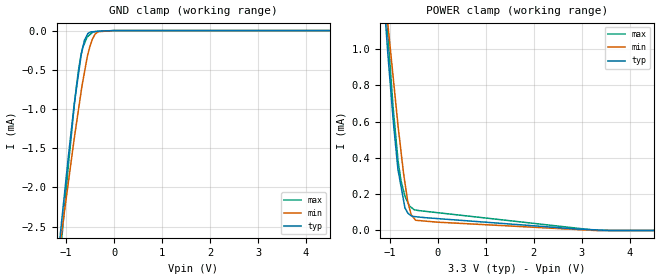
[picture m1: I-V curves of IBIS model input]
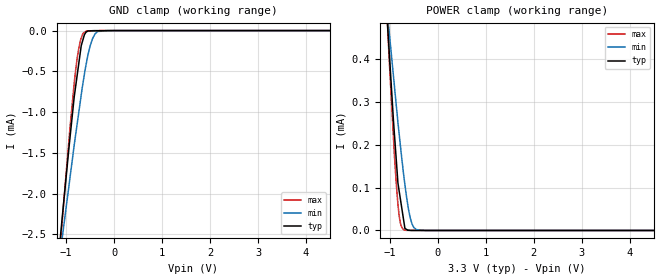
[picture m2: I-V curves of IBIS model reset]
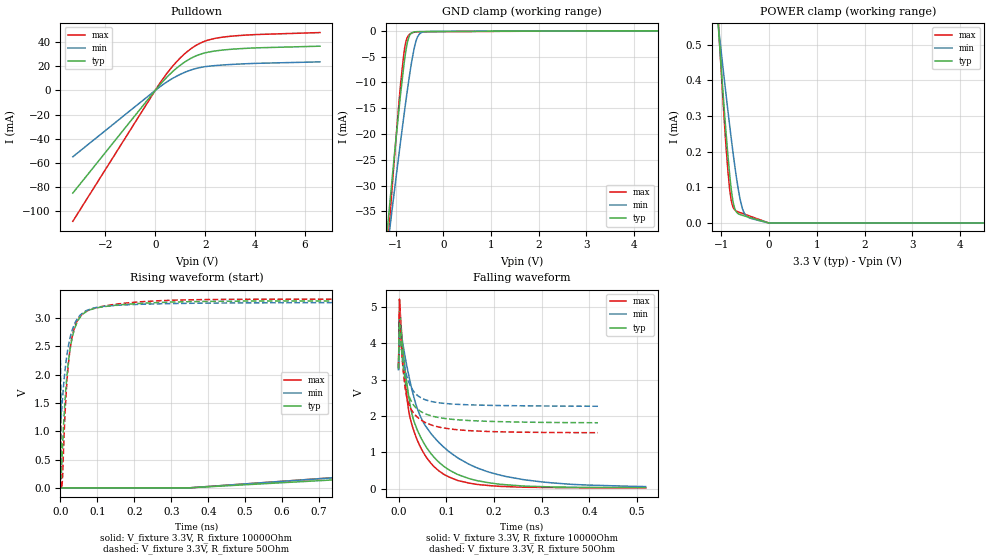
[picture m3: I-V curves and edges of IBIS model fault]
|Texas Instruments Incorporated
| 125W PurePath Digital-Input Class-D Power Stage
| Marketing part#   Digital Voltage Range   Package-type   #pins
| TAS5612LADDV   3.27V - 3.33V   DDV   44
[IBIS Ver]   3.2
[File name]   tas5612la.ibs
|SIMDE Ver   V3.0 - 201101 - Build 457
[File Rev]   1.0
[Date]   5/24/2012
[Source]
| Texas Instruments Incorporated.
| Analog-eLab Design Center, HPA
| 12500 TI Blvd
| Dallas, TX -75243
| e-mail: elab_scm_ibis@list.ti.com
[Notes]   Revision History:
| Rev 1.0: 5/24/2012
| - Initial version of the model
| - Model generated from simulations in TISPICE
| - Model matched to SPICE simulation
| - C_comp although listed in numerical order of value are
|   obtained from varying PVT conditions. For PVT conditions for
|   each specific value refer the buffer description under
|   respective [Model]. IBIS model user is responsible for using
|   appropriate C_comp to simulate for Signal Integrity.
| - Model names with a trailing _3p3 contains the model for
|   3.3V [3.27V and 3.33V].
|*  EXCEPTION:   *
|*  - For model fault, there will be a leakage current in the ground clamp  *
|*   I-V Table because of the pull-down transistor connected to pad.   *
|*  - For model clip_otw, there will be a leakage current in the ground   *
|*   clamp I-V Table because of the pull-down transistor connected to pad. *
|*  - For model input, there will be a leakage current in the power clamp   *
|*   I-V Table because of the series resistor connected to pad.   *
[Disclaimer]
| This model is designed as an aid for customers of Texas Instruments.
| TI and its licensors and suppliers make no warranties, either expressed
| or implied, with respect to this  model, including the warranties of
| merchantability or fitness for a particular purpose. The model is
| provided solely on an "as is" basis. The entire risk as to its quality
| and performance is with the customer.
[Copyright]
 (C) Copyright 2012 Texas Instruments Incorporated.All rights reserved.
|   TAS5612LA
[Component]   TAS5612LA
[Manufacturer]   TI
[Package]   |44 HTSSOP   -  DDV package
|   typ   min   max
R_pkg   0.01988   0.00761   0.02820
L_pkg   2.83543nH   1.88996nH   4.38501nH
C_pkg   0.51432pF   0.36166pF   0.71632pF
[Pin]  signal_name   model_name   R_pin   L_pin   C_pin
1   GVDD_AB   power   0.02936   5.14716nH  0.69484pF
2   VDD   power   0.02818   4.35374nH  0.68163pF
3   OC_ADJ   term   0.02761   3.69494nH  0.59541pF
4   _RESET   reset   0.02780   2.93180nH  0.42730pF
5   INPUT_A   term   0.02705   2.67858nH  0.37968pF
6   INPUT_B   term   0.02543   2.55669nH  0.37641pF
7   C_START   term   0.02324   2.39533nH  0.36233pF
8   DVDD   power   0.02065   2.21891nH  0.35477pF
9   GND   gnd   0.01893   2.09064nH  0.33358pF
10   GND   gnd   0.00713   1.79670nH  0.39618pF
11   GND   gnd   0.01384   2.26449nH  0.48602pF
12   GND   gnd   0.01381   2.27641nH  0.50323pF
13   AVDD   power   0.01424   2.33727nH  0.49485pF
14   INPUT_C   term   0.01450   2.38491nH  0.47685pF
15   INPUT_D   term   0.00761   1.88996nH  0.42531pF
16   _FAULT   fault   0.02194   2.31148nH  0.36166pF
17   _OTW   clip_otw   0.02528   2.56022nH  0.38380pF
18   _CLIP   clip_otw   0.02759   2.73531nH  0.38538pF
19   M1   input   0.02784   2.95107nH  0.42848pF
20   M2   input   0.02765   3.72216nH  0.59629pF
21   M3   input   0.02820   4.38501nH  0.67248pF
22   GVDD_CD   power   0.02952   5.32362nH  0.69982pF
23   BST_D   power   0.03232   5.58639nH  0.73537pF
24   BST_C   power   0.03291   4.81347nH  0.71048pF
25   GND   gnd   0.01175   2.94907nH  0.69322pF
26   GND   gnd   0.01186   3.22097nH  0.72361pF
27   OUT_D   term   0.01242   3.06871nH  0.71632pF
28   OUT_D   term   0.01136   2.96126nH  0.69613pF
29   PVDD_CD   power   0.01095   2.67072nH  0.66354pF
30   PVDD_CD   power   0.00938   2.40709nH  0.64271pF
31   PVDD_CD   power   0.00877   2.29583nH  0.58088pF
32   OUT_C   term   0.00921   2.31587nH  0.54265pF
33   GND   gnd   0.00969   2.46906nH  0.57388pF
34   GND   gnd   0.00969   2.46836nH  0.57309pF
35   OUT_B   term   0.00921   2.31539nH  0.54237pF
36   PVDD_AB   power   0.00878   2.29480nH  0.58034pF
37   PVDD_AB   power   0.00938   2.40544nH  0.64104pF
38   PVDD_AB   power   0.01095   2.66739nH  0.66097pF
39   OUT_A   term   0.01135   2.95115nH  0.68999pF
40   OUT_A   term   0.01242   3.06329nH  0.71322pF
41   GND   gnd   0.01186   3.16015nH  0.72229pF
42   GND   gnd   0.01174   2.94100nH  0.69314pF
43   BST_B   power   0.03289   4.77644nH  0.71393pF
44   BST_A   power   0.03229   5.53352nH  0.73759pF
[Model] term
Model_type Terminator
C_comp   1.0e-20F  1.0e-20F  1.0e-20F
|   typ   min   max
[Voltage Range]   3.3V   3.27V   3.33V
[POWER Clamp Reference]   3.3V   3.27V   3.33V
[GND Clamp Reference]   0V   0V   0V
|Ambient Temperature   25   70   0
|Junction Temperature
[Temperature Range]   27   125   0
| Models and submodels in the file (5): input (Input), reset (Input), fault (I/O_open_drain), clip_otw (Open_drain), term (Terminator)
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|   input Model
[Model]   input
Model_type   Input
Vinl = 0.8
Vinh = 1.9
|   typ   min   max
|   (nom PVT)   (fast PVT)   (slow PVT)
C_comp   2.383e-14   3.303e-15   3.538e-14
| Where nom  PVT is Nominal Process, 3.3V, 27C
|   Fast PVT is Strong Process,  3.33V, 0C
|   Slow PVT is Weak Process,   3.27V, 125C
[Voltage Range]   3.3   3.27   3.33
|Ambient Temperature   25   70   0
|Junction Temperature
[Temperature Range]   27   125   0
[Power Clamp Reference]   3.3   3.27   3.33
[GND Clamp Reference]   0   0   0
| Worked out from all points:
|   GND clamp passes 1 mA (typ) near -0.84 V on its own axis
|   POWER clamp passes 1 mA (typ) near -1.05 V on its own axis
[GND Clamp]
|   Voltage   I(typ)   I(min)   I(max)
-3.3V     -16.78mA   -13.25mA   -19.44mA
-1.112V   -2.542mA   -2.658mA   -2.794mA
-959mV    -1.641mA   -1.96mA    -1.755mA
-831.6mV  -942.3uA   -1.379mA   -961.1uA
-735.9mV  -525.1uA   -980.9uA   -482.8uA
-659.3mV  -234.9uA   -671.4uA   -227.1uA
-617.1mV  -122.2uA   -529.1uA   -162.5uA
-559.2mV  -52.14uA   -334uA     -81.21uA
-488.4mV  -16.8uA    -173.3uA   -43.59uA
-336.8mV  -9.061uA   -14.35uA   -11.13uA
-3.27mV   -64.82nA   -45.83nA   -96.5nA
6.6V      0A         0A         0A
[POWER Clamp]
|   Voltage   I(typ)   I(min)   I(max)
-3.3V     10.02mA    7.662mA    12.33mA
-1.125V   1.279mA    1.356mA    1.43mA
-1.056V   1.024mA    1.173mA    1.13mA
-1.04V    965.9uA    1.131mA    1.07mA
-932.4mV  612.3uA    848.3uA    677.8uA
-831.6mV  337.2uA    582.3uA    390.7uA
-769.2mV  246uA      439.1uA    275.6uA
-686.4mV  125uA      264.2uA    190.5uA
-627.8mV  96.81uA    160.6uA    155.5uA
-461.1mV  75.94uA    56.22uA    112.7uA
3.327V    2.999uA    0A         98nA
6.6V      0A         0A         0A
|   reset Model
[Model]   reset
Model_type   Input
Vinl = 0.8
Vinh = 1.9
|   typ   min   max
|   (nom PVT)   (fast PVT)   (slow PVT)
C_comp   2.377e-14   3.303e-15   3.567e-14
| Where nom  PVT is Nominal Process, 3.3V, 27C
|   Fast PVT is Strong Process,  3.33V, 0C
|   Slow PVT is Weak Process,   3.27V, 125C
[Voltage Range]   3.3   3.27   3.33
|Ambient Temperature   25   70   0
|Junction Temperature
[Temperature Range]   27   125   0
[Power Clamp Reference]   3.3   3.27   3.33
[GND Clamp Reference]   0   0   0
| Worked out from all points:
|   GND clamp passes 1 mA (typ) near -0.86 V on its own axis
|   POWER clamp passes 1 mA (typ) near -1.31 V on its own axis
[GND Clamp]
|   Voltage   I(typ)   I(min)   I(max)
-3.3V     -16.81mA   -13.3mA    -19.47mA
-1.154V   -2.754mA   -2.885mA   -2.878mA
-1.082V   -2.301mA   -2.549mA   -2.348mA
-1.042V   -2.056mA   -2.365mA   -2.053mA
-915.7mV  -1.294mA   -1.789mA   -1.17mA
-831.6mV  -814.3uA   -1.405mA   -645.7uA
-769.2mV  -546.4uA   -1.143mA   -338.1uA
-683.1mV  -181.5uA   -780.5uA   -86.66uA
-576.1mV  -16.4uA    -393.2uA   -4.834uA
-451.3mV  -3.585uA   -102.3uA   -1.308uA
-340.1mV  -2.374uA   -10.37uA   -20.25nA
6.6V      0A         0A         0A
[POWER Clamp]
|   Voltage   I(typ)   I(min)   I(max)
-3.3V     5.16mA     3.356mA    6.154mA
-1.049V   481.6uA    504.3uA    480.7uA
-1.016V   420.4uA    465.2uA    402.8uA
-905.8mV  225.7uA    337.7uA    176.3uA
-865.8mV  163.5uA    291.4uA    107.8uA
-829.2mV  108.5uA    249uA      57.64uA
-765.9mV  62.5uA     182.4uA    11.19uA
-689.3mV  6.826uA    109.7uA    815.9nA
-575.5mV  284.2nA    29.36uA    207.5nA
-500.3mV  47.55nA    6.964uA    115.3nA
-444.7mV  40.57nA    1.935uA    47.19nA
6.6V      0A         0A         0A
|   fault Model
[Model]   fault
Model_type   I/O_open_drain
Polarity   Inverting
Vinl = 0.8
Vinh = 1.9
Vmeas = 1.65
Vref = 3.3
Cref = 2pF
Rref = 10000
|   typ   min   max
|   (nom PVT)   (fast PVT)   (slow PVT)
C_comp   8.474e-13   8.413e-13   8.728e-13
|ON state : BUFFER OUTPUT TURNED LOW
|C_comp   8.474e-13   8.413e-13   8.728e-13
|OFF state: BUFFER IN HIGH IMPEDANCE
|C_comp   3.420e-13   2.951e-13   3.808e-13
| Where nom  PVT is Nominal Process, 3.3V, 27C
|   Fast PVT is Strong Process,  3.33V, 0C
|   Slow PVT is Weak Process,   3.27V, 125C
[Voltage Range]   3.3   3.27   3.33
|Ambient Temperature   25   70   0
|Junction Temperature
[Temperature Range]   27   125   0
[Pullup Reference]   3.3   3.27   3.33
[Pulldown Reference]   0   0   0
[Power Clamp Reference]   3.3   3.27   3.33
[GND Clamp Reference]   0   0   0
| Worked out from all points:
|   slope of the pulldown table from 0 to 0.495 V, typ, clamps not added: 42.9 ohm
|   GND clamp passes 1 mA (typ) near -0.71 V on its own axis
|   POWER clamp passes 1 mA (typ) near -1.29 V on its own axis
|   falling waveform, V_fixture 3.3V, R_fixture 10000Ohm: 20-80 % time 68.6ps typ, 114ps min, 52.7ps max; typ from 3.3 V to 0.024 V
|   rising waveform, V_fixture 3.3V, R_fixture 10000Ohm: 20-80 % time 6.39ns typ, 7.34ns min, 5.5ns max; typ from 0.018 V to 3.3 V
|   falling waveform, V_fixture 3.3V, R_fixture 50Ohm: 20-80 % time 34.3ps typ, 34.1ps min, 34.2ps max; typ from 3.3 V to 1.81 V
|   rising waveform, V_fixture 3.3V, R_fixture 50Ohm: 20-80 % time 32.9ps typ, 36.3ps min, 29.8ps max; typ from 1.8 V to 3.3 V
[Pulldown]
|   Voltage   I(typ)   I(min)   I(max)
-3.3V     -85.03mA   -54.97mA   -108.4mA
202.2mV   5.008mA    3.215mA    6.411mA
584.8mV   13.4mA     8.582mA    17.2mA
867.9mV   18.66mA    11.93mA    24.02mA
1.15V     23.07mA    14.72mA    29.81mA
1.432V    26.62mA    16.95mA    34.54mA
1.713V    29.29mA    18.6mA     38.22mA
1.995V    31.12mA    19.69mA    40.86mA
2.7V      33.45mA    21.07mA    44.13mA
3.969V    35.2mA     22.38mA    46.22mA
6.6V      36.67mA    23.68mA    47.95mA
[GND Clamp]
|   Voltage   I(typ)   I(min)   I(max)
-3.3V     -221mA     -192.5mA   -255.7mA
-1.802V   -99.82mA   -89.99mA   -119.1mA
-1.046V   -25.87mA   -32.43mA   -26.92mA
-914.1mV  -13.67mA   -22.63mA   -12.02mA
-825mV    -6.409mA   -16.25mA   -4.129mA
-785.9mV  -3.828mA   -13.55mA   -2.094mA
-742.9mV  -1.798mA   -10.69mA   -1.04mA
-654.6mV  -359.9uA   -5.418mA   -382.3uA
-594mV    -191.5uA   -2.644mA   -247.2uA
-542.8mV  -155.9uA   -1.179mA   -204.5uA
-402.6mV  -142.5uA   -182uA     -180uA
6.6V      0A         0A         0A
[POWER Clamp]
|   Voltage   I(typ)   I(min)   I(max)
-3.3V     5.287mA    3.463mA    6.313mA
-1.129V   677.4uA    632.8uA    715.7uA
-1.043V   509.2uA    527.2uA    513.6uA
-917.4mV  278.2uA    377.1uA    242.4uA
-825mV    133.2uA    271.4uA    92.66uA
-749.2mV  55.36uA    190.1uA    42.61uA
-697.1mV  33.33uA    138.8uA    34.64uA
-619.3mV  24.38uA    74.48uA    29.88uA
-542.8mV  20.92uA    34.29uA    26.13uA
-474.7mV  18.27uA    19.38uA    22.85uA
-570uV    21.98nA    19.17nA    93.78nA
6.6V      0A         0A         0A
[Ramp]
R_load = 10000
|   typ   min   max
dV/dt_r   1.96937/6.39593e-09   1.94632/7.34644e-09   1.98902/5.50141e-09
dV/dt_f   1.96937/6.89404e-11   1.94632/1.1684e-10   1.98902/5.28355e-11
[Falling Waveform]
V_fixture = 3.3V
V_fixture_min = 3.27V
V_fixture_max = 3.33V
R_fixture = 10000Ohm
|   Time   V(typ)   V(min)   V(max)
0s        3.3V       3.27V      3.33V
2ps       4.872V     4.615V     5.213V
8ps       3.997V     4.077V     3.995V
16ps      3.054V     3.472V     2.7V
26ps      2.185V     2.844V     1.86V
52ps      1.276V     1.822V     993.4mV
100ps     563.6mV    1.08V      355.2mV
152ps     258.2mV    642.1mV    139.7mV
226ps     103.4mV    329mV      52.78mV
518ps     23.99mV    53.6mV     18.42mV
[Rising Waveform]
V_fixture = 3.3V
V_fixture_min = 3.27V
V_fixture_max = 3.33V
R_fixture = 10000Ohm
|   Time   V(typ)   V(min)   V(max)
0s        17.72mV    26.13mV    14.97mV
348ps     0V         0V         0V
980ps     227.3mV    288.6mV    291.2mV
2.058ns   922.7mV    860.1mV    1.071V
4.398ns   1.828V     1.69V      2.048V
6.466ns   2.369V     2.201V     2.579V
9.208ns   2.797V     2.644V     2.961V
13.18ns   3.094V     2.983V     3.197V
16.9ns    3.208V     3.133V     3.282V
35ns      3.3V       3.27V      3.33V
[Falling Waveform]
V_fixture = 3.3V
V_fixture_min = 3.27V
V_fixture_max = 3.33V
R_fixture = 50Ohm
|   Time   V(typ)   V(min)   V(max)
0s        3.3V       3.27V      3.33V
2ps       4.574V     4.335V     4.875V
4ps       4.18V      4.08V      4.328V
8ps       3.585V     3.68V      3.513V
12ps      3.161V     3.381V     2.957V
16ps      2.854V     3.155V     2.594V
28ps      2.368V     2.749V     2.144V
50ps      2.096V     2.478V     1.862V
146ps     1.873V     2.305V     1.595V
418ps     1.81V      2.265V     1.537V
[Rising Waveform]
V_fixture = 3.3V
V_fixture_min = 3.27V
V_fixture_max = 3.33V
R_fixture = 50Ohm
|   Time   V(typ)   V(min)   V(max)
0s        1.804V     2.256V     1.534V
2ps       174.8mV    1.229V     0V
4ps       482.6mV    1.43V      0V
6ps       779.5mV    1.611V     219mV
14ps      1.694V     2.166V     1.507V
26ps      2.44V      2.646V     2.443V
42ps      2.872V     2.943V     2.897V
70ps      3.11V      3.127V     3.114V
278ps     3.273V     3.249V     3.305V
844ps     3.299V     3.268V     3.33V
